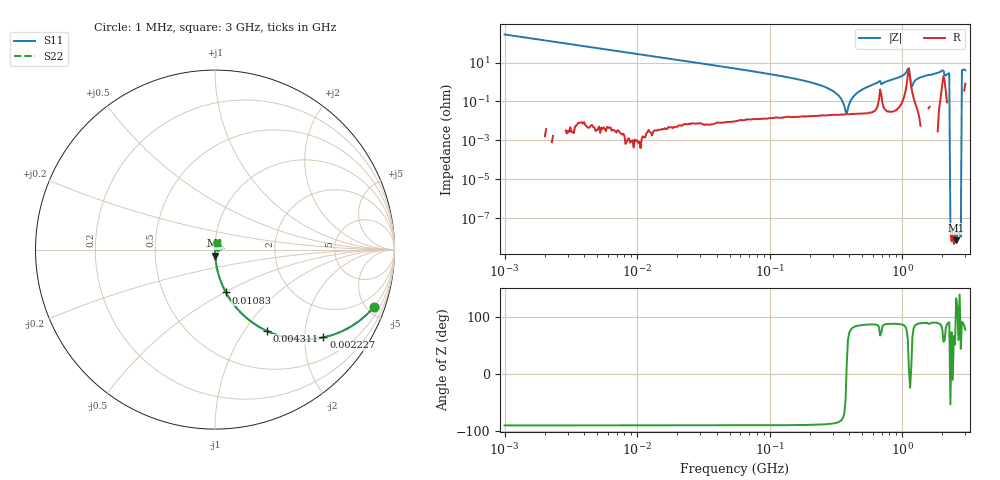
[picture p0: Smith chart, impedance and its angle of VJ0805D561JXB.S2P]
! VJ0805D561JXB
! DATE
! CORRECTED  DATA
# Hz  S  MA  R  50
!Freq	S11M	S11A	S21M	S21A	S12M	S12A	S22M	S22A
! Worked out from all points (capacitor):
!   401 points, 1 MHz to 3 GHz, reference 50 ohm
!   read as one part in series: C = 579 pF near 1.041 MHz
!   lowest |Z| = 7.34 nohm at 2.556 GHz (marker M1)
!   series resonance near 379.8 MHz, so ESL is about 300 pH
!   S11 on the Smith chart (normalised r, x): 1 MHz: 1.00, -5.50; 2.227 MHz: 1.00, -2.47; 4.311 MHz: 1.00, -1.28; 10.83 MHz: 1.00, -0.51; 3 GHz: 1.02, +0.08
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1000000  0.9399 -20.0  0.3417 70.0  0.3417 70.0  0.9399 -20.0
2226959  0.7772 -39.0  0.6293 51.0  0.6293 51.0  0.7772 -39.0
3823119  0.5839 -54.3  0.8117 35.7  0.8117 35.7  0.5839 -54.3
4310966  0.5378 -57.5  0.843 32.5  0.843 32.5  0.5378 -57.5
1.082539e7  0.2461 -75.8  0.9692 14.2  0.9692 14.2  0.2461 -75.8
1.461624e7  0.1846 -79.3  0.9828 10.6  0.9828 10.6  0.1846 -79.3
5.587962e7  0.04805 -87.1  0.9987 2.8  0.9987 2.8  0.04805 -87.1
2.094008e8  0.009132 -88.4  0.9998 0.5  0.9998 0.5  0.009132 -88.4
3.124888e8  0.002857 -85.7  0.9998 0.2  0.9998 0.2  0.002857 -85.7
3.817355e8  0.0002386 17.7  0.9998 -0.0  0.9998 -0.0  0.0002386 17.7
4.219165e8  0.001558 81.5  0.9998 -0.1  0.9998 -0.1  0.001558 81.5
4.75755e8  0.003359 85.9  0.9998 -0.2  0.9998 -0.2  0.003359 85.9
6.553423e8  0.009578 85.7  0.9993 -0.5  0.9993 -0.5  0.009578 85.7
8.005644e8  0.01195 87.8  0.9996 -0.7  0.9996 -0.7  0.01195 87.8
9.779672e8  0.01902 86.8  0.9991 -1.1  0.9991 -1.1  0.01902 86.8
1.080907e9  0.03396 75.9  0.9922 -1.9  0.9922 -1.9  0.03396 75.9
1.218836e9  0.009143 79.7  0.9984 -0.5  0.9984 -0.5  0.009143 79.7
1.347129e9  0.01624 88.5  0.9997 -0.9  0.9997 -0.9  0.01624 88.5
1.970482e9  0.03584 83.8  0.9968 -2.0  0.9968 -2.0  0.03584 83.8
2.177892e9  0.02433 86.5  0.9988 -1.4  0.9988 -1.4  0.02433 86.5
2.556106e9  0.03461 -89.6  1.001 -2.0  1.001 -2.0  0.03461 -89.6
3e9  0.03932 75.9  0.9912 -2.2  0.9912 -2.2  0.03932 75.9
